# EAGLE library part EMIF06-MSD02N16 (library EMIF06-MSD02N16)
6-Line EMI filter&ESD for SD card uQFN16 STMicroelectronics EMIF06-MSD02N16, EMI Filter & ESD Protector Source: Datasheet
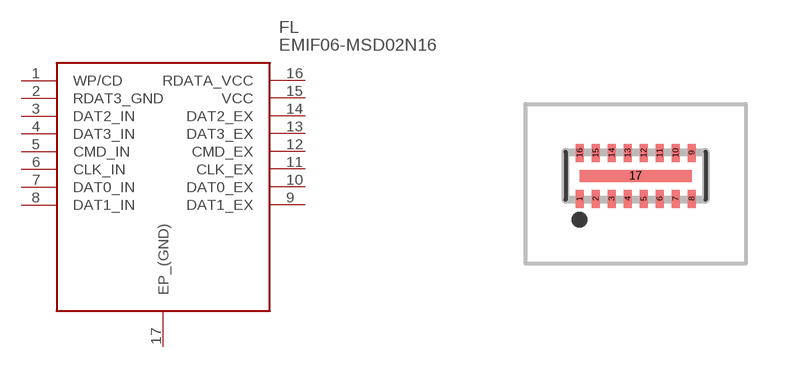
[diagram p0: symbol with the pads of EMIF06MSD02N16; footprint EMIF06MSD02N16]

Designator prefix FL

## EMIF06-MSD02N16 (Arrow_Part_Number: EMIF06-MSD02N16; Arrow_Price-Stock: https://www.arrow.com/en/products/emif06-msd02n16/stmicroelectronics?region=nac; Description: 6-Line EMI filter&ESD for SD card uQFN16 STMicroelectronics EMIF06-MSD02N16, EMI Filter & ESD Protector; Height: 0mm; Manufacturer_Name: STMicroelectronics; Manufacturer_Part_Number: EMIF06-MSD02N16; Mouser_Part_Number: 511-EMIF06-MSD02N16; Mouser_Price-Stock: https://www.mouser.co.uk/ProductDetail/STMicroelectronics/EMIF06-MSD02N16?qs=1CGoW%2F3pMwpSqVuN8kmN4Q%3D%3D)  [EMIF06MSD02N16]
1  WP/CD
2  RDAT3_GND
3  DAT2_IN
4  DAT3_IN
5  CMD_IN
6  CLK_IN
7  DAT0_IN
8  DAT1_IN
9  DAT1_EX
10  DAT0_EX
11  CLK_EX
12  CMD_EX
13  DAT3_EX
14  DAT2_EX
15  VCC
16  RDATA_VCC
17  EP_(GND)

## Footprint EMIF06MSD02N16 (pad centres in mm)
Micro QFN 3.5x1.2 16L
smd 0.2 x 0.45: 1 -1.4,-0.375; 2 -1,-0.375; 3 -0.6,-0.375; 4 -0.2,-0.375; 5 0.2,-0.375; 6 0.6,-0.375; 7 1,-0.375; 8 1.4,-0.375; 9 1.4,0.775; 10 1,0.775; 11 0.6,0.775; 12 0.2,0.775; 13 -0.2,0.775; 14 -0.6,0.775; 15 -1,0.775; 16 -1.4,0.775
smd 2.8 x 0.3: 17 0,0.2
